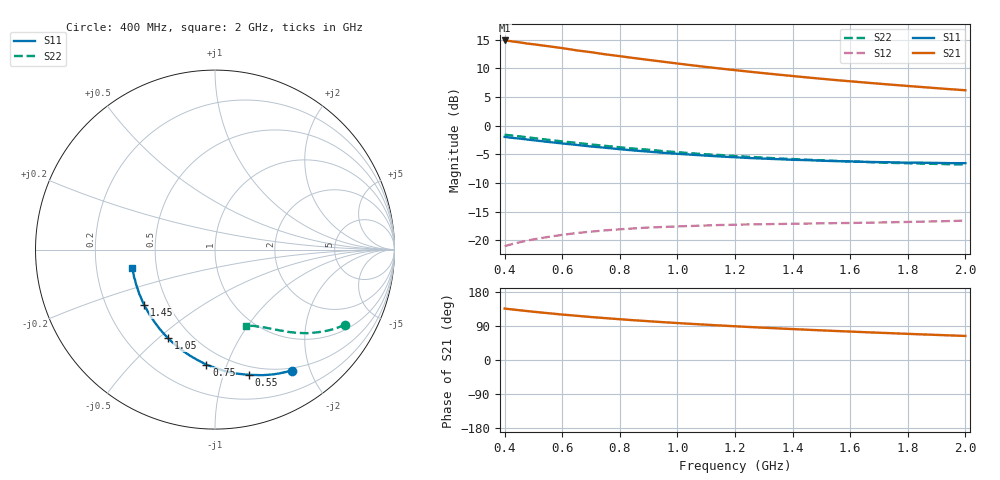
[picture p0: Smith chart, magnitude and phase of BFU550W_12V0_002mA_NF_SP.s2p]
! Filename:  P:\Prog\Test\Noise\ATS_data\Testdata_Net\06 Compressed Noise after Statistics\BFU550W_APM2013_11_D05_12p0V_002mA_NF_CM01_D.sf
! Date/Time: Tue 26/Mar/2013 16:25:25
! BFU550W_APM2013_11_D05_12p0V_1to35mA_NF_CM01_Bias2_R.sf
! Noise Parameter Data File
! BFU550W_APM2013_11_D05_12p0V_1to35mA_NF_CM01
! Date/time: Mon Mar 25 15:58:35 2013
! VAR V_out= 12.001000
! VAR I_out= 2.000000
! VAR V_in= 0.785000
! VAR I_in= 0.015595
! Device data file deembeded for feedlines and parallel
! Original file: \06 Compressed Noise after Statistics\BFU550W_APM2013_11_D05_12p0V_002mA_NF_CM01_R.sf
! Feed-files: PR019V01_070313_Feed1.s2p, PR019V01_070313_Feed2.s2p
! Parallel-file: PR019V01_070313_Par.s2p
# MHz S MA R 50
!  Freq-MHz  S11-mag  S11-arg  S21-mag  S21-arg  S12-mag  S12-arg  S22-mag  S22-arg
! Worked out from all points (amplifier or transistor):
!   37 points, 400 MHz to 2 GHz, reference 50 ohm
!   highest |S21| = 14.9 dB at 400 MHz (marker M1)
!   |S21| within 3 dB of that: start of sweep to 839.4 MHz
!   unconditionally stable (mu >= 1): nowhere
!   at 500 MHz: K = 0.28, MSG = 17.0 dB, |S12| = -19.8 dB
!   at 1.1 GHz: K = 0.59, MSG = 13.8 dB, |S12| = -17.4 dB
!   at 2 GHz: K = 0.96, MSG = 11.4 dB, |S12| = -16.5 dB
!   lowest NFmin = 0.50 dB at 420 MHz
!   S11 on the Smith chart (normalised r, x): 400 MHz: 0.46, -1.73; 550 MHz: 0.42, -1.22; 750 MHz: 0.39, -0.85; 1.05 GHz: 0.37, -0.54; 1.45 GHz: 0.37, -0.30; 2 GHz: 0.36, -0.09
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400  0.7991 -57.5  5.534 135.8  0.08922 57.8  0.8348 -30.0
420  0.7877 -60.0  5.46 133.9  0.09218 56.7  0.8245 -31.1
460  0.7681 -64.8  5.29 130.6  0.0975 54.5  0.8032 -33.1
480  0.7579 -67.0  5.193 129.1  0.0999 53.5  0.792 -34.1
500  0.7474 -69.4  5.126 127.4  0.1022 52.5  0.7813 -35.0
550  0.723 -74.8  4.935 123.6  0.1073 50.4  0.7545 -37.2
600  0.7011 -80.2  4.747 120.0  0.1119 48.3  0.7301 -39.2
650  0.6805 -84.9  4.537 116.7  0.1161 46.5  0.7091 -40.9
700  0.6593 -89.9  4.373 113.4  0.1194 45.0  0.6866 -42.7
750  0.6427 -94.3  4.19 110.5  0.1226 43.6  0.6675 -44.1
800  0.6243 -98.7  4.038 107.6  0.1252 42.4  0.6489 -45.6
850  0.6083 -102.9  3.886 104.8  0.1275 41.2  0.6318 -46.8
950  0.5811 -110.6  3.613 99.9  0.1311 39.5  0.6009 -49.3
1050  0.5591 -117.8  3.363 95.3  0.1339 38.3  0.575 -51.4
1150  0.5393 -124.7  3.147 91.0  0.1364 37.3  0.5553 -53.3
1200  0.5312 -127.7  3.051 89.0  0.1371 37.1  0.5443 -54.4
1300  0.5169 -133.8  2.87 85.2  0.1386 36.7  0.5272 -56.1
1450  0.5014 -142.1  2.636 79.9  0.1404 36.8  0.5055 -58.7
1500  0.496 -144.7  2.566 78.2  0.1411 37.0  0.4999 -59.5
1600  0.4886 -149.8  2.439 75.0  0.1421 37.5  0.4884 -61.3
1750  0.4798 -156.8  2.272 70.5  0.1443 38.8  0.4741 -63.7
2000  0.4718 -167.6  2.038 63.5  0.1489 41.6  0.4586 -68.0
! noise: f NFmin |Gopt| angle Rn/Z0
400  0.5281  0.4574  28.87  0.1829
460  0.5486  0.454  38.02  0.1802
600  0.6083  0.4608  44.99  0.1866
800  0.6546  0.4566  61.03  0.1596
1000  0.7257  0.4598  73.96  0.1588
1200  0.7418  0.4517  88.97  0.1427
1400  0.8193  0.4573  104.1  0.1134
1600  0.7254  0.4527  118.9  0.1001
1800  0.9201  0.457  132.5  0.084
2000  0.9996  0.4939  146.7  0.0638
